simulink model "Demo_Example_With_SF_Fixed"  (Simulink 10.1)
settings: Solver=FixedStepDiscrete  StartTime=0.0  StopTime=100  FixedStep=1  RelTol=1e-3

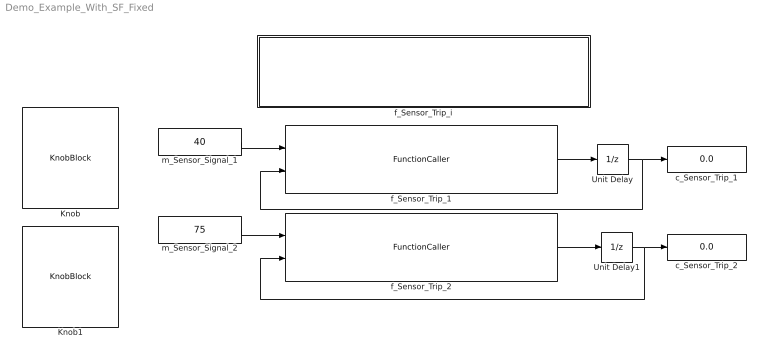
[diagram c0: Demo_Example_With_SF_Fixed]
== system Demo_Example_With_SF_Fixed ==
  Knob : KnobBlock
  Knob1 : KnobBlock
  Unit Delay : UnitDelay  SampleTime=-1  HasFrameUpgradeWarning=on
  Unit Delay1 : UnitDelay  SampleTime=-1  HasFrameUpgradeWarning=on
  c_Sensor_Trip_1 : Display
  c_Sensor_Trip_2 : Display
  f_Sensor_Trip_1 : FunctionCaller  FunctionPrototype=c_Sensor_Trip_i = f_Sensor_Trip_i(m_Sensor_Signal_i,prev_Sensor_Tripped)  InputArgumentSpecifications=int16(1), boolean(1)  OutputArgumentSpecifications=boolean(1)
  f_Sensor_Trip_2 : FunctionCaller  FunctionPrototype=c_Sensor_Trip_i = f_Sensor_Trip_i(m_Sensor_Signal_i,prev_Sensor_Tripped)  InputArgumentSpecifications=int16(1), boolean(1)  OutputArgumentSpecifications=boolean(1)
  f_Sensor_Trip_i : Subsystem
  m_Sensor_Signal_1 : Constant  Value=40  OutDataTypeStr=int16
  m_Sensor_Signal_2 : Constant  Value=75  OutDataTypeStr=int16
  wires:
  f_Sensor_Trip_1/1 -> Unit Delay/1
  f_Sensor_Trip_2/1 -> Unit Delay1/1
  m_Sensor_Signal_1/1 -> f_Sensor_Trip_1/1
  m_Sensor_Signal_2/1 -> f_Sensor_Trip_2/1
  Unit Delay/1 -> f_Sensor_Trip_1/2, c_Sensor_Trip_1/1
  Unit Delay1/1 -> f_Sensor_Trip_2/2, c_Sensor_Trip_2/1

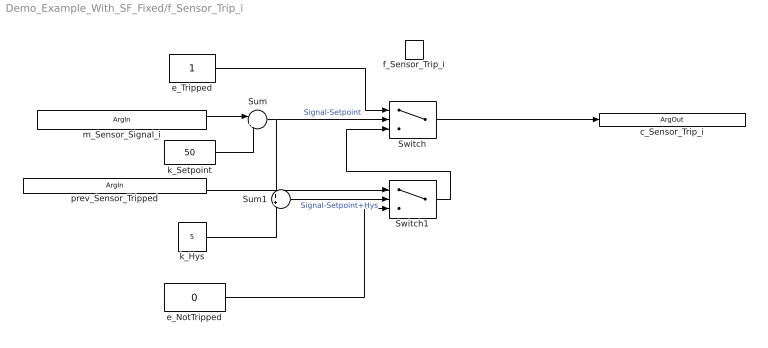
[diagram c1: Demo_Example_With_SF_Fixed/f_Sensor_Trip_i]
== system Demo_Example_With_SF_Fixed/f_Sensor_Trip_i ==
  f_Sensor_Trip_i : TriggerPort  TriggerType=function-call  IsSimulinkFunction=on  FunctionName=f_Sensor_Trip_i  FunctionVisibility=scoped  VariantControl=Variant  PortDimensions=1
  Sum : Sum  Inputs=|+-  AccumDataTypeStr=int16
  Sum1 : Sum  AccumDataTypeStr=int16
  Switch : Switch  OutDataTypeStr=boolean
  Switch1 : Switch  OutDataTypeStr=boolean
  e_NotTripped : Constant  Value=0  OutDataTypeStr=boolean
  e_Tripped : Constant  OutDataTypeStr=boolean
  k_Hys : Constant  Value=5  OutDataTypeStr=int16
  k_Setpoint : Constant  Value=50  OutDataTypeStr=int16
  m_Sensor_Signal_i : ArgIn  OutDataTypeStr=int16  ArgumentName=m_Sensor_Signal_i
  prev_Sensor_Tripped : ArgIn  Port=2  OutDataTypeStr=boolean  ArgumentName=prev_Sensor_Tripped
  c_Sensor_Trip_i : ArgOut  OutDataTypeStr=boolean  ArgumentName=c_Sensor_Trip_i
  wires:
  m_Sensor_Signal_i/1 -> Sum/1
  Sum/1 -> Switch/2, Sum1/1  "Signal-Setpoint"
  e_Tripped/1 -> Switch/1
  Switch/1 -> c_Sensor_Trip_i/1
  Switch1/1 -> Switch/3
  k_Hys/1 -> Sum1/2
  Sum1/1 -> Switch1/2  "Signal-Setpoint+Hys"
  e_NotTripped/1 -> Switch1/3
  k_Setpoint/1 -> Sum/2
  prev_Sensor_Tripped/1 -> Switch1/1
